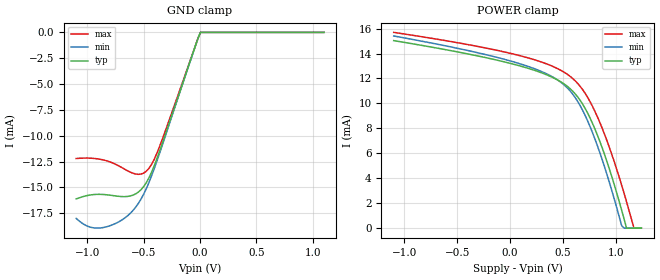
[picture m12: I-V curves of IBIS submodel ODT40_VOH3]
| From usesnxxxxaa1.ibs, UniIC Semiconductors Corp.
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|   Submodel ODT40_VOH3
[Submodel] ODT40_VOH3
Submodel_type Dynamic_clamp
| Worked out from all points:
|   GND clamp passes 1 mA (typ) near -0.03 V on its own axis
[GND_clamp]
|Voltage   I(typ)   I(min)   I(max)
-1.1V     -16.12mA   -18.01mA   -12.21mA
-962mV    -15.72mA   -18.89mA   -12.18mA
-870mV    -15.68mA   -18.91mA   -12.32mA
-778mV    -15.79mA   -18.62mA   -12.63mA
-617mV    -15.83mA   -17.48mA   -13.54mA
-548mV    -15.46mA   -16.55mA   -13.74mA
-479mV    -14.57mA   -15.16mA   -13.45mA
-433mV    -13.59mA   -13.95mA   -12.82mA
-364mV    -11.65mA   -11.85mA   -11.17mA
-65mV     -2.07mA    -2.079mA   -2.023mA
4mV       79.17nA    663.9nA    14.11nA
1.1V      0A         0A         0A
[POWER_clamp]
|Voltage   I(typ)   I(min)   I(max)
-1.1V     15.04mA    15.41mA    15.7mA
-372mV    13.92mA    14.19mA    14.67mA
111mV     12.96mA    13.13mA    13.79mA
387mV     12.14mA    12.19mA    13.03mA
571mV     11.15mA    10.96mA    12.14mA
686mV     9.927mA    9.429mA    11.09mA
801mV     7.955mA    7.153mA    9.367mA
916mV     5.306mA    4.269mA    6.984mA
1.054V    1.431mA    189.6uA    3.438mA
1.1V      0A         0A         2.119mA
1.17V     0A         0A         0A
1.24V     0A         0A         0A
